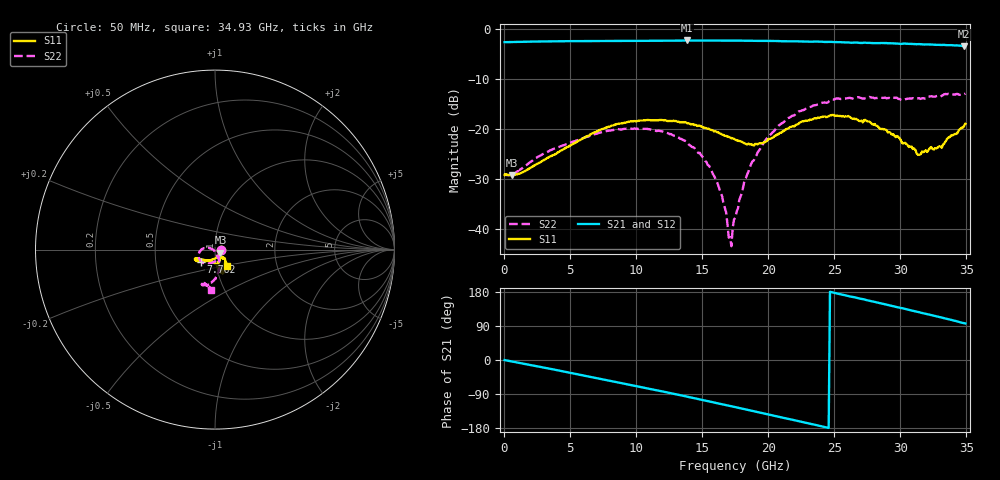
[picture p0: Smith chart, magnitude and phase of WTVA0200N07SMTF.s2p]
! 50 ohm 2-Port S-parameters measured by Modelithics Inc support@modelithics.com  Tampa, FL USA 813-866-6335 (February 2024)
! Smiths Interconnect,  2dB P/N: WTVA0200N07SMTF, Temperature: -25 C
! Board: 10 mil Rogers 4350B, Mounting Pad Dimensions: Length: 15 mils, Width: 25 mils, Gap: 40 mils.
# Hz S RI R 50
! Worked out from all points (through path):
!   352 points, 50 MHz to 34.93 GHz, reference 50 ohm
!   highest |S21| = -2.22 dB at 13.83 GHz (marker M1); lowest = -3.4 dB at 34.83 GHz (marker M2)
!   group delay of S21, straight-line fit = 21 ps
!   lowest |S11| = -29.2 dB at 598 MHz (marker M3), VSWR 1.07, Z = 53.1 - j1.76 ohm
!   |S11| at or under -10 dB: start of sweep to end of sweep
!   |S22| runs from -43.4 to -12.9 dB; largest |S21 - S12| = 0.0082
!   S11 on the Smith chart (normalised r, x): 50 MHz: 1.07, -0.00; 7.762 GHz: 0.84, -0.11; 34.93 GHz: 1.13, -0.21
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5e7  0.0348 -0.0012  0.744 -0.00276  0.7432 -0.00324  0.0362 -0.00114
5.98e8  0.0306 -0.0166  0.746 -0.0477  0.7452 -0.0477  0.0308 -0.0176
5.8715e9  -0.0478 -0.0639  0.5869 -0.4872  0.5856 -0.4872  -0.0264 -0.0761
7.762e9  -0.0801 -0.0669  0.4608 -0.6106  0.4596 -0.6102  -0.0574 -0.0769
1.1742e10  -0.111 -0.0545  0.1178 -0.7598  0.1154 -0.7592  -0.0914 -0.0321
1.38315e10  -0.104 -0.0505  -0.0884 -0.7692  -0.09 -0.7682  -0.0754 0.00214
1.612e10  -0.0767 -0.0538  -0.3099 -0.7073  -0.3116 -0.7055  -0.0288 0.00868
1.68165e10  -0.0645 -0.0564  -0.3744 -0.6742  -0.3764 -0.672  -0.0147 0.0015
1.70155e10  -0.0608 -0.0577  -0.3918 -0.6642  -0.3937 -0.6622  -0.0081 -0.00153
1.72145e10  -0.0569 -0.0581  -0.4092 -0.6541  -0.4106 -0.6522  -0.00355 -0.00576
1.7314e10  -0.0556 -0.0589  -0.4181 -0.6487  -0.4194 -0.6467  -0.00282 -0.0099
1.7513e10  -0.0523 -0.0586  -0.4356 -0.6367  -0.4372 -0.6343  -0.00172 -0.0129
1.82095e10  -0.0386 -0.0611  -0.4912 -0.5918  -0.4925 -0.5894  0.0103 -0.029
1.9702e10  -0.00536 -0.0741  -0.5986 -0.4815  -0.599 -0.4796  0.0248 -0.0705
2.13935e10  0.0239 -0.0979  -0.6839 -0.3288  -0.6844 -0.3255  0.0204 -0.1261
2.33835e10  0.041 -0.119  -0.7409 -0.1351  -0.7404 -0.1324  -0.0062 -0.1723
2.607e10  0.0394 -0.1299  -0.7264 0.1439  -0.7248 0.1464  -0.0566 -0.1973
2.91545e10  0.0171 -0.0921  -0.5907 0.423  -0.5875 0.4256  -0.069 -0.1941
3.1443e10  0.0302 -0.0466  -0.4172 0.5774  -0.413 0.5791  -0.049 -0.1986
3.31345e10  0.0473 -0.045  -0.2615 0.6466  -0.2561 0.6476  -0.0241 -0.2148
3.4826e10  0.0666 -0.0853  -0.085 0.6732  -0.0783 0.673  -0.0188 -0.2238
3.49255e10  0.0683 -0.0908  -0.0765 0.6756  -0.0698 0.6752  -0.0206 -0.2265
